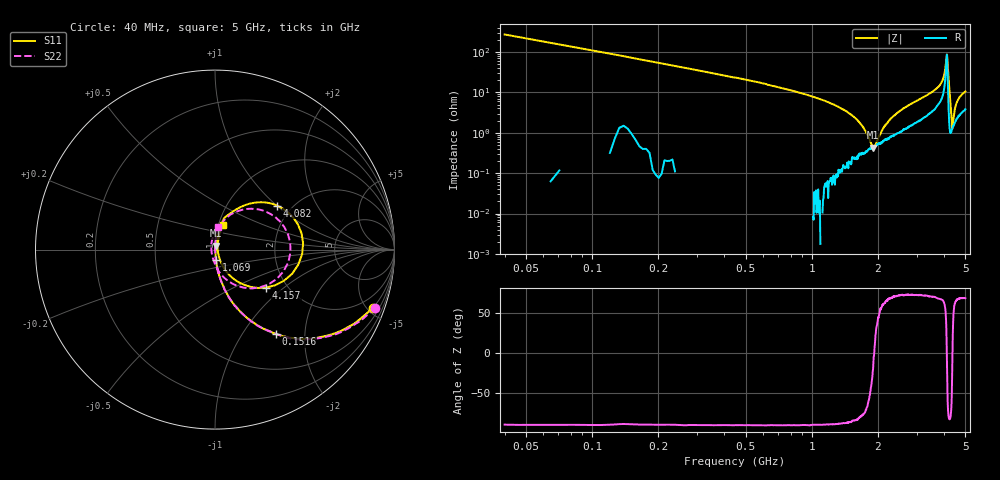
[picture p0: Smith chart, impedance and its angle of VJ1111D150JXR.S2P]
! VJ1111D150JXR
! DATE 02/16/2022  10:08
! CAPACITORS MOUNTED IN SERIES ON 25 MIL THICK MICROSTRIP SUBSTRATE
# GHz  S  MA  R  50.00
!  FREQ  S11M  S11A  S21M  S21A  S12M  S12A  S22M  S22A
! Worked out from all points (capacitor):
!   801 points, 40 MHz to 5 GHz, reference 50 ohm
!   read as one part in series: C = 14.5 pF near 64.8 MHz
!   lowest |Z| = 428 mohm at 1.906 GHz (marker M1)
!   series resonance near 1.924 GHz, so ESL is about 470 pH
!   S11 on the Smith chart (normalised r, x): 40 MHz: 1.04, -5.40; 151.6 MHz: 1.01, -1.43; 1.069 GHz: 1.00, -0.12; 4.082 GHz: 1.68, +1.01; 4.157 GHz: 1.57, -0.76; 5 GHz: 1.05, +0.29
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0.04  0.9356 -20.3  0.3458 69.5  0.3445 69.5  0.9479 -20.0
0.1516  0.5788 -54.2  0.8107 35.2  0.8135 36.5  0.5827 -53.9
0.35  0.2848 -73.2  0.9582 17.1  0.9627 16.8  0.2883 -73.0
0.8708  0.08895 -83.7  0.995 6.3  0.9998 6.2  0.08971 -84.0
1.0692  0.05859 -84.5  0.9951 4.8  0.9998 4.7  0.05875 -85.9
1.5032  0.01052 -73.9  0.9952 2.8  0.9998 2.6  0.01133 -85.7
1.5714  0.005877 -57.0  0.9942 2.4  0.9997 2.3  0.005366 -87.1
1.6334  0.003304 15.9  0.9934 2.3  0.9988 2.1  0.0005236 -9.5
1.6954  0.00664 59.4  0.9932 2.1  0.9989 1.9  0.004731 83.8
1.7822  0.01314 74.5  0.993 1.8  0.9975 1.6  0.01162 87.4
1.9062  0.02214 79.1  0.9914 1.4  0.9972 1.2  0.02062 88.4
2.52  0.06242 81.0  0.9815 -0.1  0.987 -0.4  0.06003 86.7
3.3508  0.119 77.7  0.956 -2.5  0.9616 -2.5  0.1093 80.5
3.822  0.1956 71.4  0.9138 -4.7  0.9207 -4.8  0.1541 74.8
4.0824  0.4245 35.3  0.6649 -11.5  0.6683 -11.6  0.3674 32.7
4.1196  0.4922 4.2  0.5306 8.4  0.533 8.2  0.421 -1.9
4.1568  0.3552 -36.5  0.7916 21.9  0.7967 21.9  0.2974 -46.7
4.1754  0.2577 -50.0  0.89 18.0  0.8943 17.9  0.2136 -62.9
4.2932  0.01493 13.6  0.9746 5.0  0.9802 4.9  0.02025 -179.7
4.3676  0.0517 69.8  0.9722 2.7  0.9777 2.6  0.04676 113.8
4.4668  0.07944 73.4  0.9683 0.8  0.9731 0.7  0.07395 97.4
5  0.1439 72.5  0.9388 -2.8  0.9443 -3.0  0.1289 82.7
